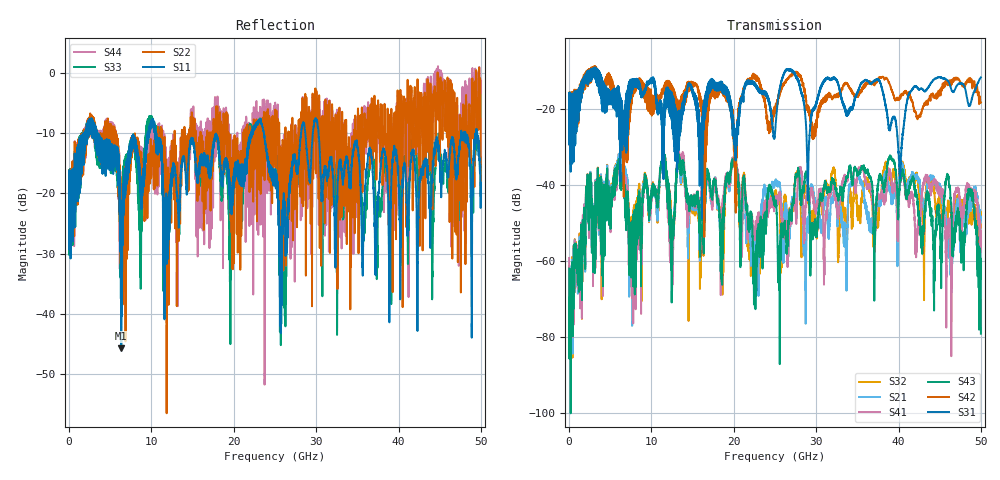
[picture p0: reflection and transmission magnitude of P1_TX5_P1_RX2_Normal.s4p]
!Keysight Technologies,N5225B,MY57041031,A.13.20.10
!Date: Friday, May 31, 2019 11:15:50
!Correction: S11(Full 4 Port(1,2,3,4))
!S12(Full 4 Port(1,2,3,4))
!S13(Full 4 Port(1,2,3,4))
!S14(Full 4 Port(1,2,3,4))
!S21(Full 4 Port(1,2,3,4))
!S22(Full 4 Port(1,2,3,4))
!S23(Full 4 Port(1,2,3,4))
!S24(Full 4 Port(1,2,3,4))
!S31(Full 4 Port(1,2,3,4))
!S32(Full 4 Port(1,2,3,4))
!S33(Full 4 Port(1,2,3,4))
!S34(Full 4 Port(1,2,3,4))
!S41(Full 4 Port(1,2,3,4))
!S42(Full 4 Port(1,2,3,4))
!S43(Full 4 Port(1,2,3,4))
!S44(Full 4 Port(1,2,3,4))
!S4P File: Measurements: <S11,S12,S13,S14>,
!<S21,S22,S23,S24>,
!<S31,S32,S33,S34>,
!<S41,S42,S43,S44>:
# Hz S  dB  R 50.0
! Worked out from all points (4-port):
!   5000 points, 10 MHz to 50 GHz, reference 50 ohm
!   strongest paths, dB at 10 MHz, 12.51 GHz, 25.01 GHz, 37.51 GHz, 50 GHz:
!     S31: -19.4, -23.1, -26.2, -12.3, -11.7
!     S42: -19.4, -16.4, -19.7, -12.4, -18.4
!     S43: -62.1, -55.8, -44.8, -40.1, -79.2
!     S41: -59.3, -68.0, -44.1, -42.7, -55.1
!     S21: -66.5, -57.1, -39.5, -44.9, -49.5
!     S32: -61.3, -55.5, -42.4, -50.4, -48.4
!   lowest |S11| = -45.7 dB at 6.34 GHz (marker M1), VSWR 1.01, Z = 49.6 - j0.3 ohm
!   |S11| at or under -10 dB: 3.502 GHz to 9.556 GHz (6.054 GHz wide, 92.7 % of centre); 10.5 GHz to 22.11 GHz (11.6 GHz wide, 71.2 % of centre); 30.29 GHz to 47.6 GHz (17.31 GHz wide, 44.4 % of centre)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
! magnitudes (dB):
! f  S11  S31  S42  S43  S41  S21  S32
! 10 MHz  -19.8  -19.4  -19.4  -62.1  -59.3  -66.5  -61.3
! 6.34 GHz  -45.7  -20.2  -30.5  -40.9  -40.6  -38.0  -38.3
! 19.99 GHz  -18.8  -24.4  -25.0  -33.8  -33.4  -33.4  -34.1
! 22.59 GHz  -9.0  -13.3  -11.9  -68.7  -52.5  -56.1  -65.9
! 39.07 GHz  -20.5  -24.0  -14.4  -32.7  -38.0  -42.0  -39.3
! 48.82 GHz  -25.6  -18.2  -12.9  -41.7  -42.3  -45.5  -47.4
! 50 GHz  -18.2  -11.7  -18.4  -79.2  -55.1  -49.5  -48.4
